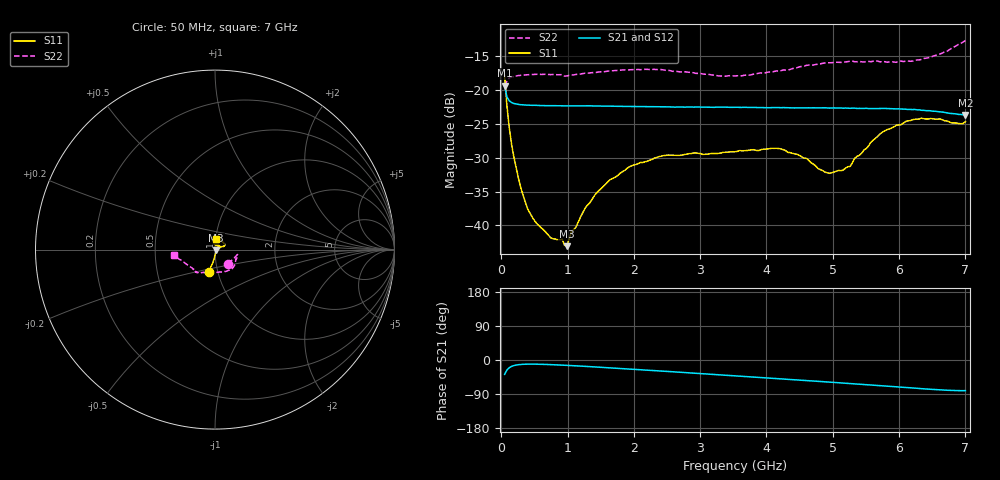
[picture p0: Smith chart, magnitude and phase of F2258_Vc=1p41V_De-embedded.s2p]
! Integrated Device Technology
! Corporate Headquarters
! 6024 Silver Creek Valley Road
! San Jose, CA 95138  USA
! Phone:  1-408-284-8200
! Toll Free:  1-800-223-1366
! Webpage:  http://www.idt.com/
! Timing and RF Division
! 515 Groton Road, Suite 102
! Westford, MA 01886-6024
! Device:  F2258
! Description: Voltage Variable RF Attenuator
! Frequency:  50.0 -  6000.00 MHz
! Package:  3x3 mm Thin QFN Plastic Package: 16 pin
! Ports:  2 RF, 2 DC
!  Pin  1  = NC
!  Pin  2  = NC
!  Pin  3  = RF2  = Port 2
!  Pin  4  = GND
!  Pin  5  = Vdd
!  Pin  6  = NC
!  Pin  7  = VCTRL
!  Pin  8  = NC
!  Pin  9  = GND
!  Pin 10  = RF1  = Port 1
!  Pin 11  = NC
!  Pin 12  = NC
!  Pin 13  = NC
!  Pin 14  = NC
!  Pin 15  = NC
!  Pin 16  = NC
! Vcntrl:  1.410 Volts
! Vdd:  +3.300 Volts
! Current:  1.164 mA
! Data:  The device was measured on a the F2258 evaluation board which has
!  individual transmission lines to the RF pins.  Data was collected
!  using a calibrated network analyzer.  The evaluation board was
!  de-embedded using a TRL calibration technique.
!  The reference plane is the edge of the package pin.
! Misc:  SN 10
!  Action Tracker AT0285
! Date Measured:  2014-12-10
! Date:  2016-01-13  MJV
! Note:
!  Integrated Device Technology supplies this data as a sample of measured
!  data at the package pin for this product.  Your particular data for this
!  product may vary.
!  Data was taken at 25 degrees C.
!  Integrated Device Technology reserves the right to change this data at anytime.
!Freq_(GHz)  S11M_(dB)  S11P_(deg)  S21M_(dB)  S21P_(deg)  S12M_(dB)  S12P_(deg)  S22M_(dB)  S22P_(deg)
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# GHz S dB R 50
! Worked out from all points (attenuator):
!   201 points, 50 MHz to 7 GHz, reference 50 ohm
!   highest |S21| = -19.32 dB at 50 MHz (marker M1); lowest = -23.7 dB at 7 GHz (marker M2)
!   lowest |S11| = -43.1 dB at 988.2 MHz (marker M3), VSWR 1.01, Z = 50.6 - j0.331 ohm
!   |S11| at or under -10 dB: start of sweep to end of sweep
!   |S22| runs from -19.4 to -12.6 dB; largest |S21 - S12| = 0.00049
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0.05  -17.84 -106.1  -19.32 -37.9  -19.33 -37.9  -19.41 -47.1
0.08475  -22.31 -99.7  -21.00 -26.4  -21.01 -26.5  -18.63 -24.0
0.15425  -27.97 -93.4  -21.83 -16.9  -21.85 -16.9  -18.05 -14.7
0.29325  -34.40 -82.3  -22.15 -11.8  -22.15 -11.8  -17.80 -12.4
0.3975  -37.56 -73.7  -22.21 -10.9  -22.22 -10.9  -17.72 -13.0
0.745  -41.85 -36.1  -22.30 -12.2  -22.30 -12.2  -17.71 -19.3
0.91875  -42.04 -10.3  -22.32 -13.6  -22.34 -13.6  -17.71 -23.7
0.98825  -43.08 -27.8  -22.33 -14.1  -22.33 -14.1  -17.90 -25.0
1.05775  -40.91 -16.1  -22.32 -14.7  -22.35 -14.7  -17.77 -26.3
1.2315  -38.08 -2.1  -22.33 -16.4  -22.34 -16.4  -17.54 -29.9
1.6485  -33.20 9.4  -22.37 -20.9  -22.39 -20.9  -17.16 -38.0
1.9265  -31.36 18.5  -22.42 -23.9  -22.42 -23.9  -17.00 -43.2
2.37825  -29.84 30.2  -22.45 -28.8  -22.44 -28.8  -16.96 -52.2
3.525  -29.12 82.3  -22.54 -41.8  -22.51 -41.9  -17.90 -88.6
4.18525  -28.64 101.9  -22.58 -49.4  -22.56 -49.5  -17.18 -112.0
4.7065  -30.94 91.1  -22.61 -55.4  -22.57 -55.5  -16.28 -122.9
4.94975  -32.31 70.8  -22.65 -58.3  -22.62 -58.4  -15.96 -125.3
5.15825  -31.82 49.7  -22.67 -60.8  -22.63 -60.9  -15.85 -127.3
5.71425  -26.45 20.3  -22.70 -67.6  -22.69 -67.6  -15.82 -132.0
5.85325  -25.74 20.8  -22.73 -69.4  -22.73 -69.4  -15.83 -134.7
6.33975  -24.13 28.5  -22.98 -75.7  -22.99 -75.7  -15.45 -146.8
7  -24.66 83.7  -23.66 -80.9  -23.68 -80.8  -12.65 -172.4
